[IBIS Ver]  2.1
[File Name] sprm027.ibs
[File Rev]  0.1
[Date]   February 21, 2001
[Source]   IBIS Model Generated from PACED
[Disclaimer]   Please be aware that in the absence of a written agreement
|   Texas Instruments(TI) assumes no liability for:
|   (1) The accuracy of the IBIS models provided to your company
|   (2) The proper functioning of these Models in your design
|   or for any resulting applications; or
|   (3)Infringement of patents, copyrights or intellectual
|   property rights resulting from your use of these models.
|   TI provides IBIS Models as a service to our customers and
|   therefore reserves the right to limit distribution of the
|   Models.
[Copyright]   Property of Texas Instruments Incorporated.
|   Unauthorized reproduction and/or distribution is strictly.
|   prohibited.
|   This product is protected under copyright law and trade
|   secret law as an unpublished work.
|   Created 1999,(C) Copyright 1999-2000,
|   Texas Instruments Incorporated., All Rights Reserved.
|   These commodities are under the U.S.
|   Government distribution license control. As such,they
|   are not to be re-exported without the prior approval of
|   the U.S.Department of Commerce.
[Component]   c6202_GLS
[Manufacturer]   Texas Instruments
[Package]
|Variable   Typ   Min   Max
R_pkg   0.07725   0.03872   0.1717
L_pkg   1.18E-09  5.92E-10  2.62E-09
C_pkg   2.60E-13  1.28E-13  5.40E-13
[Pin] signal_name   model_name   R_pin   L_pin   C_pin
B10   CLKIN   UIT293   0.07231   1.10E-09   2.48E-13
Y18   CLKOUT1   UOT254   0.05834   8.86E-10   2.21E-13
AB19  CLKOUT2   UOT254   0.1224   1.87E-09   4.19E-13
B12   CLKMODE0   UIT293   0.06676   1.02E-09   2.22E-13
Y5   TMS   UIT293   0.05804   8.85E-10   2.21E-13
AA4   TDO   UOT254   0.1016   1.55E-09   3.54E-13
Y4   TDI   UIT293   0.0589   8.98E-10   2.12E-13
AB2   TCK   UIT293   0.1523   2.32E-09   4.91E-13
AA3   TRST   UIT293   0.08289   1.26E-09   2.94E-13
AA5   EMU1   UIT285_UOT254   0.08663   1.33E-09   3.08E-13
AB4   EMU0   UIT285_UOT254   0.1098   1.68E-09   3.78E-13
J3   RESET   UIT293   0.04191   6.39E-10   1.32E-13
K2   NMI   UIT293   0.07207   1.10E-09   2.38E-13
U2   EXT_INT7   UIT293   0.07566   1.15E-09   2.62E-13
U3   EXT_INT6   UIT293   0.04749   7.14E-10   1.75E-13
W1   EXT_INT5   UIT293   0.1289   1.96E-09   4.24E-13
V2   EXT_INT4   UIT293   0.08616   1.31E-09   2.90E-13
V1   IACK   UOT254   0.1187   1.81E-09   3.87E-13
R3   INUM3   UOT254   0.04594   6.97E-10   1.62E-13
T1   INUM2   UOT254   0.1029   1.57E-09   3.42E-13
T2   INUM1   UOT254   0.06501   9.90E-10   2.18E-13
T3   INUM0   UOT254   0.04339   6.64E-10   1.36E-13
Y2   PD   UOT254   0.09297   1.42E-09   2.94E-13
C8   XCLKIN   UIT293   0.03872   5.92E-10   1.30E-13
A8   XFCLK   UOT254   0.1015   1.54E-09   3.41E-13
C13   XD31   UIT285_UOT254   0.04331   6.62E-10   1.61E-13
A13   XD30   UIT285_UOT254   0.09336   1.42E-09   3.08E-13
C14   XD29   UIT285_UOT254   0.05875   8.97E-10   1.90E-13
B14   XD28   UIT285_UOT254   0.07149   1.10E-09   2.36E-13
B15   XD27   UIT285_UOT254   0.07422   1.13E-09   2.46E-13
C15   XD26   UIT285_UOT254   0.03891   5.93E-10   1.30E-13
A15   XD25   UIT285_UOT254   0.07588   1.16E-09   2.56E-13
B16   XD24   UIT285_UOT254   0.08721   1.33E-09   2.97E-13
C16   XD23   UIT285_UOT254   0.04412   6.70E-10   1.57E-13
A17   XD22   UIT285_UOT254   0.0895   1.37E-09   2.99E-13
B17   XD21   UIT285_UOT254   0.06658   1.02E-09   2.25E-13
C17   XD20   UIT285_UOT254   0.04793   7.25E-10   1.82E-13
B18   XD19   UIT285_UOT254   0.08663   1.33E-09   3.08E-13
A19   XD18   UIT285_UOT254   0.1098   1.68E-09   3.78E-13
C18   XD17   UIT285_UOT254   0.05804   8.85E-10   2.21E-13
B19   XD16   UIT285_UOT254   0.1016   1.55E-09   3.54E-13
C19   XD15   UIT285_UOT254   0.0589   8.98E-10   2.12E-13
B20   XD14   UIT285_UOT254   0.08289   1.26E-09   2.94E-13
A21   XD13   UIT285_UOT254   0.1523   2.32E-09   4.91E-13
C21   XD12   UIT285_UOT254   0.09297   1.42E-09   2.94E-13
D20   XD11   UIT285_UOT254   0.04842   7.33E-10   1.81E-13
B22   XD10   UIT285_UOT254   0.122   .86E-09   4.05E-13
D21   XD9   UIT285_UOT254   0.07149   1.09E-09   2.39E-13
E20   XD8   UIT285_UOT254   0.04426   6.75E-10   1.49E-13
E21   XD7   UIT285_UOT254   0.08616   1.31E-09   2.90E-13
D22   XD6   UIT285_UOT254   0.1289   1.96E-09   4.24E-13
F20   XD5   UIT285_UOT254   0.04749   7.14E-10   1.75E-13
F21   XD4   UIT285_UOT254   0.07566   1.15E-09   2.62E-13
E22   XD3   UIT285_UOT254   0.1187   1.81E-09   3.87E-13
G20   XD2   UIT285_UOT254   0.04339   6.64E-10   1.36E-13
G21   XD1   UIT285_UOT254   0.06501   9.90E-10   2.18E-13
G22   XD0   UIT285_UOT254   0.1029   1.57E-09   3.42E-13
D2   XCE3   UOT254   0.07129   1.09E-09   2.39E-13
B1   XCE2   UOT254   0.1343   2.05E-09   4.43E-13
D3   XCE1   UOT254   0.04818   7.32E-10   1.81E-13
C2   XCE0   UOT254   0.06903   1.06E-09   2.19E-13
C5   XBE3XA5   UIT285_UOT254   0.05834   8.86E-10   2.21E-13
A4   XBE2XA4   UIT285_UOT254   0.1224   1.87E-09   4.19E-13
B5   XBE1XA3   UIT285_UOT254   0.09008   1.37E-09   3.18E-13
C6   XBE0XA2   UIT285_UOT254   0.0484   7.27E-10   1.82E-13
A6   XOE   UOT254   0.1136   1.73E-09   3.79E-13
C7   XRE   UOT254   0.04439   6.69E-10   1.62E-13
B7   XWEXWAIT   UOT254   0.06635   1.01E-09   2.25E-13
C9   XCS   UIT293   0.0571   8.71E-10   1.83E-13
B6   XAS   UIT285_UOT254   0.07658   1.16E-09   2.58E-13
B9   XCNTL   UIT293   0.07059   1.08E-09   2.27E-13
B8   XWR   UIT285_UOT254   0.06216   9.47E-10   2.03E-13
C4   XRDY   UIT285_UOT254   0.06538   9.96E-10   2.31E-13
B4   XBLAST   UIT285_UOT254   0.102   .56E-09   3.49E-13
A10   XBOFF   UIT293   0.1051   1.61E-09   3.32E-13
A2   XHOLD   UIT285_UOT254   0.154   .36E-09   5.00E-13
B3   XHOLDA   UIT285_UOT254   0.1136   1.73E-09   3.89E-13
Y21   CE3   UOT254   0.06903   1.06E-09   2.19E-13
W20   CE2   UOT254   0.04818   7.32E-10   1.81E-13
AA22  CE1   UOT254   0.1343   2.05E-09   4.43E-13
W21   CE0   UOT254   0.07129   1.09E-09   2.39E-13
V20   BE3   UOT254   0.04421   6.75E-10   1.49E-13
V21   BE2   UOT254   0.08607   1.31E-09   2.90E-13
W22   BE1   UOT254   0.1109   1.69E-09   3.69E-13
U20   BE0   UOT254   0.04769   7.15E-10   1.75E-13
H20   EA21   UIT285_UOT254   0.04594   6.97E-10   1.62E-13
H21   EA20   UIT285_UOT254   0.07421   1.13E-09   2.57E-13
H22   EA19   UIT285_UOT254   0.09568   1.46E-09   3.18E-13
J20   EA18   UIT285_UOT254   0.04167   6.38E-10   1.32E-13
J21   EA17   UIT285_UOT254   0.07597   1.16E-09   2.50E-13
K21   EA16   UIT285_UOT254   0.0686   1.05E-09   2.27E-13
K20   EA15   UIT285_UOT254   0.04465   6.76E-10   1.57E-13
K22   EA14   UIT285_UOT254   0.09949   1.51E-09   3.40E-13
L21   EA13   UIT285_UOT254   0.06585   1.00E-09   2.17E-13
L20   EA12   UIT285_UOT254   0.0406   6.20E-10   1.30E-13
L22   EA11   UIT285_UOT254   0.1717   2.62E-09   5.40E-13
M20   EA10   UIT285_UOT254   0.0406   6.20E-10   1.30E-13
M21   EA9   UIT285_UOT254   0.06609   1.01E-09   2.17E-13
N22   EA8   UIT285_UOT254   0.09972   1.51E-09   3.40E-13
N20   EA7   UIT285_UOT254   0.04474   6.77E-10   1.57E-13
N21   EA6   UIT285_UOT254   0.07207   1.10E-09   2.38E-13
P21   EA5   UIT285_UOT254   0.07902   1.20E-09   2.59E-13
P20   EA4   UIT285_UOT254   0.04191   6.39E-10   1.32E-13
R22   EA3   UIT285_UOT254   0.09547   1.45E-09   3.19E-13
R21   EA2   UIT285_UOT254   0.07413   1.13E-09   2.57E-13
Y6   ED31   UIT285_UOT254   0.04793   7.25E-10   1.82E-13
AA6   ED30   UIT285_UOT254   0.06658   1.02E-09   2.25E-13
AB6   ED29   UIT285_UOT254   0.0895   1.37E-09   2.99E-13
Y7   ED28   UIT285_UOT254   0.04412   6.70E-10   1.57E-13
AA7   ED27   UIT285_UOT254   0.08721   1.33E-09   2.97E-13
AB8   ED26   UIT285_UOT254   0.07588   1.16E-09   2.56E-13
Y8   ED25   UIT285_UOT254   0.03891   5.93E-10   1.30E-13
AA8   ED24   UIT285_UOT254   0.07422   1.13E-09   2.46E-13
AA9   ED23   UIT285_UOT254   0.07149   1.10E-09   2.36E-13
Y9   ED22   UIT285_UOT254   0.05875   8.97E-10   1.90E-13
AB10  ED21   UIT285_UOT254   0.09336   1.42E-09   3.08E-13
Y10   ED20   UIT285_UOT254   0.04331   6.62E-10   1.61E-13
AA10  ED19   UIT285_UOT254   0.09586   1.47E-09   3.15E-13
AA11  ED18   UIT285_UOT254   0.06676   1.02E-09   2.22E-13
Y11   ED17   UIT285_UOT254   0.05997   9.17E-10   1.96E-13
AB12  ED16   UIT285_UOT254   0.1646   2.52E-09   5.19E-13
Y12   ED15   UIT285_UOT254   0.04013   6.13E-10   1.28E-13
AA12  ED14   UIT285_UOT254   0.06598   1.01E-09   2.17E-13
AA13  ED13   UIT285_UOT254   0.07231   1.10E-09   2.48E-13
Y13   ED12   UIT285_UOT254   0.04419   6.66E-10   1.61E-13
AB13  ED11   UIT285_UOT254   0.1051   1.61E-09   3.32E-13
Y14   ED10   UIT285_UOT254   0.0571   8.71E-10   1.83E-13
AA14  ED9   UIT285_UOT254   0.07059   1.08E-09   2.27E-13
AA15  ED8   UIT285_UOT254   0.06216   9.47E-10   2.03E-13
Y15   ED7   UIT285_UOT254   0.03872   5.92E-10   1.30E-13
AB15  ED6   UIT285_UOT254   0.1015   1.54E-09   3.41E-13
AA16  ED5   UIT285_UOT254   0.06635   1.01E-09   2.25E-13
Y16   ED4   UIT285_UOT254   0.04439   6.69E-10   1.62E-13
AB17  ED3   UIT285_UOT254   0.1136   1.73E-09   3.79E-13
AA17  ED2   UIT285_UOT254   0.07658   1.16E-09   2.58E-13
Y17   ED1   UIT285_UOT254   0.0484   7.27E-10   1.82E-13
AA18  ED0   UIT285_UOT254   0.09008   1.37E-09   3.18E-13
T21   ARE   UOT254   0.08092   1.23E-09   2.74E-13
R20   AOE   UOT254   0.04613   6.97E-10   1.62E-13
T22   AWE   UOT254   0.1027   1.57E-09   3.42E-13
T20   ARDY   UIT293   0.04343   6.60E-10   1.43E-13
AA19  SDA10   UOT254   0.102   .56E-09   3.49E-13
AB21  SDCAS_SSADS   UOT254   0.154   .36E-09   5.00E-13
Y19   SDRAS_SSOE   UOT254   0.06538   9.96E-10   2.31E-13
AA20  SDWE_SSWE   UOT254   0.1136   1.73E-09   3.89E-13
V22   HOLD   UIT293   0.1191   1.81E-09   3.89E-13
U21   HOLDA   UOT254   0.07593   1.15E-09   2.62E-13
D1   TOUT0   UOT254   0.1109   1.69E-09   3.69E-13
E2   TINP0   UIT293   0.08607   1.31E-09   2.90E-13
F2   TOUT1   UOT254   0.07593   1.15E-09   2.62E-13
F3   TINP1   UIT293   0.04769   7.15E-10   1.75E-13
V3   DMAC3   UOT254   0.04426   6.75E-10   1.49E-13
W2   DMAC2   UOT254   0.07149   1.09E-09   2.39E-13
AA1   DMAC1   UOT254   0.122   .86E-09   4.05E-13
W3   DMAC0   UOT254   0.04842   7.33E-10   1.81E-13
K3   CLKS0   UIT293   0.04474   6.77E-10   1.57E-13
L2   CLKR0   UIT285_UOT254   0.06609   1.01E-09   2.17E-13
K1   CLKX0   UIT285_UOT254   0.09972   1.51E-09   3.40E-13
M2   DR0   UIT293   0.06585   1.00E-09   2.17E-13
M3   DX0   UOT254   0.0406   6.20E-10   1.30E-13
M1   FSR0   UIT285_UOT254   0.1717   2.62E-09   5.40E-13
L3   FSX0   UIT285_UOT254   0.0406   6.20E-10   1.30E-13
E1   CLKS1   UIT293   0.1191   1.81E-09   3.89E-13
G2   CLKR1   UIT285_UOT254   0.08092   1.23E-09   2.74E-13
G3   CLKX1   UIT285_UOT254   0.04343   6.60E-10   1.43E-13
H1   DR1   UIT293   0.09547   1.45E-09   3.19E-13
H2   DX1   UOT254   0.07413   1.13E-09   2.57E-13
H3   FSR1   UIT285_UOT254   0.04613   6.97E-10   1.62E-13
G1   FSX1   UIT285_UOT254   0.1027   1.57E-09   3.42E-13
N1   CLKS2   UIT293   0.09949   1.51E-09   3.40E-13
N2   CLKR2   UIT285_UOT254   0.0686   1.05E-09   2.27E-13
N3   CLKX2   UIT285_UOT254   0.04465   6.76E-10   1.57E-13
R2   DR2   UIT293   0.07421   1.13E-09   2.57E-13
R1   DX2   UOT254   0.09568   1.46E-09   3.18E-13
P3   FSR2   UIT285_UOT254   0.04167   6.38E-10   1.32E-13
P2   FSX2   UIT285_UOT254   0.07597   1.16E-09   2.50E-13
| End of package information
[Component]   UIT293
[Manufacturer]   Texas Instruments
[Package]
|   typ   min   max
R_pkg   0   0   0
L_pkg   0   0   0
C_pkg   0   0   0
[Pin]   signal_name   model_name   R_pin   L_pin   C_pin
   1   A   UIT293   0   0   0
[Component]   UIT285_UOT212
[Manufacturer]   Texas Instruments
[Package]
|   typ   min   max
R_pkg   0   0   0
L_pkg   0   0   0
C_pkg   0   0   0
[Pin]   signal_name   model_name   R_pin   L_pin   C_pin
   1   Y   UIT285_UOT212   0   0   0
[Component]   UIT286
[Manufacturer]   Texas Instruments
[Package]
|   typ   min   max
R_pkg   0   0   0
L_pkg   0   0   0
C_pkg   0   0   0
[Pin]   signal_name   model_name   R_pin   L_pin   C_pin
   1   Y   UIT286   0   0   0
[Component]   UIT293_UOT212
[Manufacturer]   Texas Instruments
[Package]
|   typ   min   max
R_pkg   0   0   0
L_pkg   0   0   0
C_pkg   0   0   0
[Pin]   signal_name   model_name   R_pin   L_pin   C_pin
   1   Y   UIT293_UOT212   0   0   0
[Component]   UOT212
[Manufacturer]   Texas Instruments
[Package]
|   typ   min   max
R_pkg   0   0   0
L_pkg   0   0   0
C_pkg   0   0   0
[Pin]   signal_name   model_name   R_pin   L_pin   C_pin
   1   Y   UOT212   0   0   0
[Component]   UIT293_UPT219
[Manufacturer]   Texas Instruments
[Package]
|   typ   min   max
R_pkg   0   0   0
L_pkg   0   0   0
C_pkg   0   0   0
[Pin]   signal_name   model_name   R_pin   L_pin   C_pin
   1   A   UIT293_UPT219   0   0   0
[Component]   UOT254
[Manufacturer]   Texas Instruments
[Package]
|   typ   min   max
R_pkg   0   0   0
L_pkg   0   0   0
C_pkg   0   0   0
[Pin]   signal_name   model_name   R_pin   L_pin   C_pin
   1   Y   UOT254   0   0   0
[Component]   UIT285_UOT254
[Manufacturer]   Texas Instruments
[Package]
|   typ   min   max
R_pkg   0   0   0
L_pkg   0   0   0
C_pkg   0   0   0
[Pin]   signal_name   model_name   R_pin   L_pin   C_pin
   1   Y   UIT285_UOT254   0   0   0
| Models and submodels in the file (8): UIT293 (Input), UIT285_UOT212 (I/O), UIT286 (Input), UIT293_UOT212 (I/O), UOT212 (3-state), UIT293_UPT219 (Input), UOT254 (3-state), UIT285_UOT254 (I/O)
